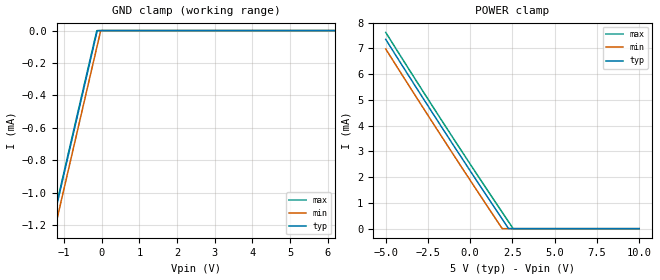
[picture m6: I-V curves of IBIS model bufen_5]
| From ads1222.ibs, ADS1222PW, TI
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|   bufen_5 Model
[Model]   bufen_5
Model_type   Input
Vinl = 1
Vinh = 4
|   typ   min   max
|   (nom PVT)   (fast PVT)   (slow PVT)
|C_comp from frequency sweep method (F= 8MHz)
|Average
C_comp   1.020e-15   8.637e-16   1.225e-15
|C_comp from LC tank measurement(L=1nH)
|Average
|Resonant Frequency(Hz)   1.000e+12   1.000e+12   1.000e+12
|C_comp   2.536e-17   2.536e-17   2.536e-17
[Model spec]
Vinl   1   0.9   1.1
Vinh   4   3.6   4.4
| Where nom  PVT is Nominal Process, 5V, 25C
|   Fast PVT is Strong Process,  5.5V, -40C
|   Slow PVT is Weak Process,   4.5V, 85C
[Voltage Range]   5   4.5   5.5
|Ambient Temperature   25   85   -40
|Junction Temperature
[Temperature Range]   25   85   -40
[Power Clamp Reference]   5   4.5   5.5
[GND Clamp Reference]   0   0   0
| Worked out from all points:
|   GND clamp passes 1 mA (typ) near -1.12 V on its own axis
[GND Clamp]
|   Voltage   I(typ)   I(min)   I(max)
-5V       -4.997mA   -5.083mA   -4.996mA
-1.728V   -1.621mA   -1.712mA   -1.609mA
-1.25V    -1.136mA   -1.228mA   -1.125mA
-132.5mV  -13.61uA   -105.6uA   -1.964uA
-121.5mV  -2.622uA   -94.61uA   0A
-27.5mV   -257.5nA   -723.6nA   0A
-18.5mV   -173.2nA   0A         0A
10V       0A         0A         0A
[POWER Clamp]
|   Voltage   I(typ)   I(min)   I(max)
-5V       7.354mA    6.98mA     7.625mA
-1.728V   3.985mA    3.617mA    4.246mA
1.894V    371.6uA    2.888uA    636.8uA
2.27V     3.332uA    0A         269.3uA
2.541V    928.6nA    0A         4.889uA
10V       0A         0A         0A
